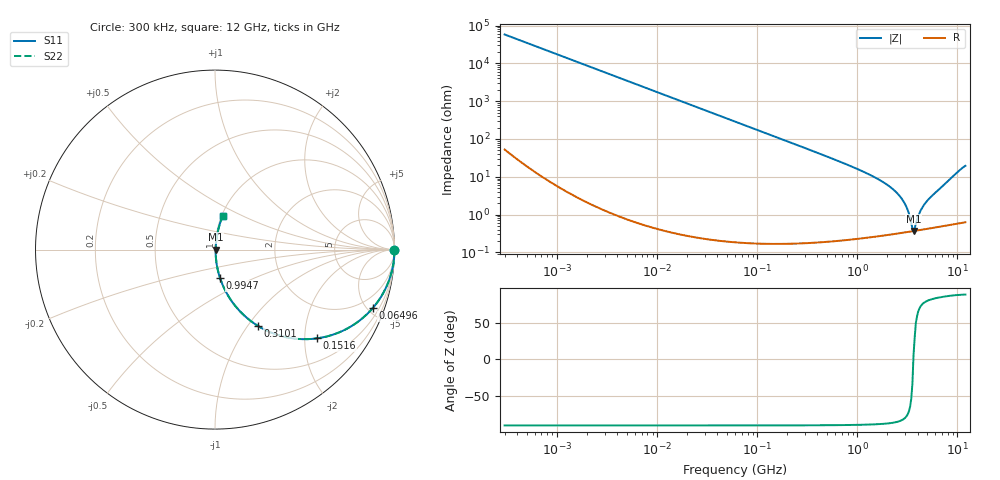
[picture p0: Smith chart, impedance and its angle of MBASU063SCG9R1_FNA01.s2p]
! MBASU063SCG9R1_FNA01  S-PARAMETER MODEL  ( Standard Model )
! Model Generated by TAIYO YUDEN Corporation (http://www.ty-top.com)
! Version 1.0
! TAIYO YUDEN Control No. 230609
! Copyright(c) 2023 TAIYO YUDEN CO.,LTD. All Rights Reserved.
! Product Description (link to TY-COMPAS)
! https://ds.yuden.co.jp/TYCOMPAS/or/detail?pn=MBASU063SCG9R1CFNA01&u=M
! Products Name : Multilayer Ceramic Capacitors
! Characteristics :
!  Capacitance : 9.1 [pF] , Rated Voltage : 50 [V] , TCC : CG / C0G
!  Case Size : 0.6 x 0.3 / 0.024 x 0.012 [mm/inch] , Thickness : 0.3 / 0.012 [mm/inch]
!  (Conditions: Temperature = 25 [degC] , DC Bias Voltage = 0 [V])
! External Node Assignments :
!  1  o---| |---o  2
! GND o---------o GND
! Frequency Range : 0.3MHz  -  12000MHz  [ 401 STEP ]
# MHZ S RI R 50
! Freq[MHz].  S11 Real  S11 Imag  S21 Real  S21 Imag  S12 Real  S12 Imag  S22 Real  S22 Imag
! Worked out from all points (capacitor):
!   401 points, 300 kHz to 12 GHz, reference 50 ohm
!   read as one part in series: C = 9.14 pF near 316.3 kHz
!   lowest |Z| = 369 mohm at 3.643 GHz (marker M1)
!   series resonance near 3.629 GHz, so ESL is about 210 pH
!   S11 on the Smith chart (normalised r, x): 300 kHz: open; 64.96 MHz: 1.00, -5.36; 151.6 MHz: 1.00, -2.29; 310.1 MHz: 1.00, -1.11; 994.7 MHz: 1.00, -0.32; 12 GHz: 1.01, +0.39
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0.3  1 -0.00172  4.53e-06 0.00172  4.53e-06 0.00172  1 -0.00172
1.769972  0.9999 -0.0102  0.000106 0.0102  0.000106 0.0102  0.9999 -0.0102
10.44266  0.9964 -0.0598  0.0036 0.0598  0.0036 0.0598  0.9964 -0.0598
26.39317  0.9775 -0.1482  0.0225 0.1482  0.0225 0.1482  0.9775 -0.1482
60  0.8936 -0.308  0.1064 0.308  0.1064 0.308  0.8936 -0.308
64.96309  0.8775 -0.3275  0.1225 0.3275  0.1225 0.3275  0.8775 -0.3275
151.6462  0.5676 -0.4947  0.4324 0.4947  0.4324 0.4947  0.5676 -0.4947
310.0777  0.2377 -0.4241  0.7623 0.4241  0.7623 0.4241  0.2377 -0.4241
353.9943  0.1927 -0.3926  0.8073 0.3926  0.8073 0.3926  0.1927 -0.3926
555.3718  0.0872 -0.2789  0.9128 0.2789  0.9128 0.2789  0.0872 -0.2789
994.7115  0.0276 -0.1571  0.9724 0.1571  0.9724 0.1571  0.0276 -0.1571
2088.533  0.00601 -0.0554  0.994 0.0554  0.994 0.0554  0.00601 -0.0554
2514.07  0.00443 -0.0359  0.9956 0.0359  0.9956 0.0359  0.00443 -0.0359
2870.14  0.00383 -0.0227  0.9962 0.0227  0.9962 0.0227  0.00383 -0.0227
3107.553  0.00365 -0.015  0.9964 0.015  0.9964 0.015  0.00365 -0.015
3454.93  0.0036 -0.00486  0.9964 0.00486  0.9964 0.00486  0.0036 -0.00486
3642.919  0.00365 0.000411  0.9963 -0.000411  0.9963 -0.000411  0.00365 0.000411
3841.137  0.00376 0.00437  0.9962 -0.00437  0.9962 -0.00437  0.00376 0.00437
4385.161  0.00414 0.0136  0.9959 -0.0136  0.9959 -0.0136  0.00414 0.0136
5006.236  0.00472 0.0229  0.9953 -0.0229  0.9953 -0.0229  0.00472 0.0229
9708.23  0.0206 0.1208  0.9794 -0.1208  0.9794 -0.1208  0.0206 0.1208
12000  0.0422 0.1857  0.9578 -0.1857  0.9578 -0.1857  0.0422 0.1857
